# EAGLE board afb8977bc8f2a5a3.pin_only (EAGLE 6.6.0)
REV: A

Size 50.8 x 22.86 mm. Coordinates in mm from the lower left corner, seen from the top.
Outline: 2.54,0 48.26,0 arc90 50.8,2.54 50.8,20.32 arc90 48.26,22.86 2.54,22.86 arc90 0,20.32 0,13.97 0.51,13.46 0.51,9.4 0,8.89 0,2.54 arc90 2.54,0
Copper layers (1*16): Top 0.035mm / dielectric 1.5mm / Bottom 0.035mm
Design rules "adafruit *": minimum track width 8mil, minimum drill 15.5mil, track to track 8mil, track to pad 8mil, pad to pad 8mil, via to via 8mil, smd to smd 8mil, copper to edge 10mil, drill to drill 8mil, minimum pad ring 10mil, minimum via ring 8mil, stop-mask expansion 2mil, vias tented up to drill 20mil, thermal gap 10mil
Holes 2.54 mm at 48.26,20.32 48.26,2.54
tRestrict: area 21.3,6.9 to 21.7,9.7; area 22.1,12.1 to 27.1,12.4; area 26.5,9.7 to 27.1,12.2

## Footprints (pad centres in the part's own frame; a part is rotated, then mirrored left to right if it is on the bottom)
0603-NO = smd 1.1 x 1: 1 -0.85,0; 2 0.85,0
0805-NO = smd 1.24 x 1.5: 1 -0.95,0; 2 0.95,0
CHIPLED_0805_NOOUTLINE = smd 1.2 x 1.2: A 0,-1.05; C 0,1.05
SOD-123 = smd 1.4 x 1.4: A 1.85,0; C -1.85,0
1X16_ROUND = drill 1 pad 1.676: 1 -19.05,0; 2 -16.51,0; 3 -13.97,0; 4 -11.43,0; 5 -8.89,0; 6 -6.35,0; 7 -3.81,0; 8 -1.27,0; 9 1.27,0; 10 3.81,0; 11 6.35,0; 12 8.89,0; 13 11.43,0; 14 13.97,0; 15 16.51,0; 16 19.05,0
1X01_ROUND = drill 1 pad 1.676: 1 0,0
1X12_ROUND = drill 1 pad 1.676: 1 -13.97,0; 2 -11.43,0; 3 -8.89,0; 4 -6.35,0; 5 -3.81,0; 6 -1.27,0; 7 1.27,0; 8 3.81,0; 9 6.35,0; 10 8.89,0; 11 11.43,0; 12 13.97,0
1X03_ROUND = drill 1 pad 1.676: 1 -2.54,0; 2 0,0; 3 2.54,0
KMR2 = smd 1 x 1: 1 2,0.8; 2 2,-0.8; 3 -2,0.8; 4 -2,-0.8
TESTPOINT_ROUND_1.5MM = smd 1.5 x 1.5: P$1 0,0
SOT23-5 = smd 0.55 x 1.2: 1 -0.95,-1.3; 2 0,-1.3; 3 0.95,-1.3; 4 0.95,1.3; 5 -0.95,1.3
RFMHCW_SMT = smd 1.5 x 1: 1P 8.1,-7; 2P 8.1,-5; 3P 8.1,-3; 4P 8.1,-1; 5P 8.1,1; 6P 8.1,3; 7P 8.1,5; 8P 8.1,7; 9P -8.1,7; 10P -8.1,5; 11P -8.1,3; 12P -8.1,1; 13P -8.1,-1; 14P -8.1,-3; 15P -8.1,-5; 16P -8.1,-7
TQFN48_7MM = smd 0.25 x 0.75: 1 -2.75,-3.475; 2 -2.25,-3.475; 3 -1.75,-3.475; 4 -1.25,-3.475; 5 -0.75,-3.475; 6 -0.25,-3.475; 7 0.25,-3.475; 8 0.75,-3.475; 9 1.25,-3.475; 10 1.75,-3.475; 11 2.25,-3.475; 12 2.75,-3.475; 25 2.75,3.475; 26 2.25,3.475; 27 1.75,3.475; 28 1.25,3.475; 29 0.75,3.475; 30 0.25,3.475; 31 -0.25,3.475; 32 -0.75,3.475; 33 -1.25,3.475; 34 -1.75,3.475; 35 -2.25,3.475; 36 -2.75,3.475 | smd 0.75 x 0.25: 13 3.475,-2.75; 14 3.475,-2.25; 15 3.475,-1.75; 16 3.475,-1.25; 17 3.475,-0.75; 18 3.475,-0.25; 19 3.475,0.25; 20 3.475,0.75; 21 3.475,1.25; 22 3.475,1.75; 23 3.475,2.25; 24 3.475,2.75; 37 -3.475,2.75; 38 -3.475,2.25; 39 -3.475,1.75; 40 -3.475,1.25; 41 -3.475,0.75; 42 -3.475,0.25; 43 -3.475,-0.25; 44 -3.475,-0.75; 45 -3.475,-1.25; 46 -3.475,-1.75; 47 -3.475,-2.25; 48 -3.475,-2.75 | smd 4.7 x 4.7: THERMAL 0,0
MOUNTINGHOLE_2.5_PLATED = drill 2.5 pad 3.2: P$1 0,0
FIDUCIAL_1MM = smd 1 x 1: 1 0,0
JSTPH2 = smd 1 x 4.6: 1 -1,-3.7; 2 1,-3.7 | smd 1.6 x 3.4: NC1 -3.4,1.5; NC2 3.4,1.5
XTAL3215 = smd 1.1 x 1.9: P$1 1.2,0; P$2 -1.2,0
4UCONN_20329_V2 = smd 1 x 2: BASE@1 -0.75,-2; BASE@2 0.75,-2 | smd 0.4 x 1.35: D+ 0,0.775; D- -0.65,0.775; GND 1.3,0.775; ID 0.65,0.775; VBUS -1.3,0.775 | drill 0.8 pad 1.2 offset: SPRT@1 -3.3,0.9; SPRT@2 3.3,0.9 | drill 0.9 pad 2.5 square: SPRT@3 -3.6,-1.9; SPRT@4 3.6,-1.9 | hole 0.7: -1.95,0; 1.95,0
U.FL = smd 2.2 x 1.05: 1 0,1.375; 2 0,-1.375 | smd 0.8 x 1: 3 1.525,0

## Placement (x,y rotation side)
C1  1uF  [0603-NO]  17.78,11.81 90 top
C2  22pF  [0603-NO]  17.65,7.49 90 top
C3  10µF  [0805-NO]  11.43,11.18 270 top
C4  22pF  [0603-NO]  16.38,7.49 90 top
C5  10uF  [0805-NO]  28.96,17.53 90 top
C6  10µF  [0805-NO]  8.09,12.96 90 top
C7  1uF  [0603-NO]  16.4,11.86 90 top
C8  10µF  [0805-NO]  13.86,11.62 270 top
C9  10uF  [0805-NO]  49.53,8.76 270 top
C14  1uF  [0603-NO]  10.72,4.34 0 top
CHG  ORANGE  [CHIPLED_0805_NOOUTLINE]  2.41,5.59 270 top
D1  MBR120  [SOD-123]  17.78,18.67 180 top
JP1  [1X16_ROUND]  25.4,1.27 180 top
JP2  [1X01_ROUND]  49.53,5.08 0 top
JP3  [1X12_ROUND]  30.48,21.59 0 top
JP5  [1X03_ROUND]  49.53,15.24 90 top
L  RED  [CHIPLED_0805_NOOUTLINE]  2.65,17.36 90 top
R1  100k  [0603-NO]  15.62,16.13 90 top
R2  1K  [0603-NO]  6.1,4.32 0 top
R3  100k  [0603-NO]  22.1,18.67 0 top
R6  100K  [0603-NO]  22.48,17.4 180 top
R7  2.2K  [0603-NO]  5.71,20.95 270 top
R8  10K\  [0603-NO]  13.84,4.32 180 top
SW1  SPST_TACT-KMR2  [KMR2]  9.4,6.48 180 top
TP1  [TESTPOINT_ROUND_1.5MM]  15.37,5.33 0 bottom
TP2  [TESTPOINT_ROUND_1.5MM]  17.91,5.33 0 bottom
U2  AP2112K-3.3  [SOT23-5]  18.16,15.49 180 top
U3  MCP73831T-2ACI/OT  [SOT23-5]  13.84,7.75 180 top
U4  RFM69HCW  [RFMHCW_SMT]  39.12,11.43 0 top
U$4  ATSAMD21G18_QFN  [TQFN48_7MM]  24.13,9.65 0 top
U$7  [ADAFRUIT_3.5MM]  24.26,15.49 0 top
U$9  [FEATHERLOGO]  30.35,6.48 0 bottom
U$12  [ADAFRUIT_3.5MM]  3.05,13.34 180 bottom
U$13  [PCBFEAT-REV-040]  4.32,4.95 0 bottom
U$31  MOUNTINGHOLE2.5  [MOUNTINGHOLE_2.5_PLATED]  2.54,20.32 270 top
U$32  MOUNTINGHOLE2.5  [MOUNTINGHOLE_2.5_PLATED]  2.54,2.54 270 top
U$34  FIDUCIAL""  [FIDUCIAL_1MM]  10.79,20.07 270 top
U$35  FIDUCIAL""  [FIDUCIAL_1MM]  46.4,0.77 270 top
X1  JSTPH  [JSTPH2]  10.79,19.3 0 top
X2  32.768  [XTAL3215]  17.78,4.83 0 top
X3  microUSB  [4UCONN_20329_V2]  4.45,11.43 270 top
X4  uFL  [U.FL]  45.59,5.08 180 bottom

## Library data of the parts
C1-C7 C9 C14 CHG D1 JP1-JP3 JP5 L R1-R3 R6-R8 TP1 TP2 U2-U4 U$4 U$7 U$9 U$12 U$13 X1 X3 X4 = microbuilder
C8 = microbuilder; COMPANY: ADAFRUIT INDUSTRIES; DRAWN: KTOWN; REV: A
SW1 = adafruit
U$31 U$32 U$34 U$35 = microbuilder; BOM: EXCLUDE
X2 = adafruit2

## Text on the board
tPlace: BAT | En | USB | 13 | 12 | 11 | ~ | 10 | ~ | ~ | 9 | 6 | ~ | 5 | SCL | SDA | #13 | RFM9x LoRa | RFM9x / LoRa | Reset | adafruit! | CHG | Feather M0 | RST | 3V | ARf | GND | A0 | A1 | A2 | A3 | A4 | A5 | SCK | MOS | MIS | RX0 | TX1 | io1
bPlace: 21 | 20 | 3.7/4.2V / LiPoly Batt / µUSB charge | En | 13 | 12 | 6 | ~ | 5 | SCL | SDA | BAT | USB | 11~ | 10~ | 9~ | D2 | Feather M0 / RFM9x LoRa Radio | D3 | Node# | ATSAMD21G18 3.3V | D5 | RF Radio uses: / MISO/MOSI/SCK / 4 RST,3 IRQ,8 CS | Ant. | swclk | swdio | SCK | 24 | MOSI | 23 | MISO | Freq | +20dBm | RST | 3V | ARf | GND | A0 | A1 | A2 | A3 | A4 | A5 | 22 | RX | TX | io1 | 0 | 1

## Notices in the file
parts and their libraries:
microbuilder: This work is placed in the public domain, and may be freely used for commercial and non-commercial work with the following conditions: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
